| IBIS file stm32u535_545_ufbga100_smps.ibs
[IBIS ver] 4.2
[File name] stm32u535_545_ufbga100_smps.ibs
[File Rev] rev1.0
[Date]  11-09-2023
[Source] Data Created at STMicroelectronics
[Notes]  File originated from ELDO simulations.
[Disclaimer]  This information is for modeling purpose only and is
   not guaranteed. The information is subject to change without
   notice.
[Copyright] Copyright 2023 STMicroelectronics Inc.
|   Component stm32u535_545_ufbga100_smps
[Component] stm32u535_545_ufbga100_smps
[Manufacturer] STMicroelectronics
[Package]
| variable   typ   min   max
R_pkg  0  NA  NA
L_pkg  0  NA  NA
C_pkg  0  NA  NA
[Pin]   signal_name   model_name
A1  PB9  io8_100m_hslv_i2c_ft
A2  PE0  io8_100m_hslv_ft
A3  PH3-BOOT0  io8_100m_ft
A4  PB7  io8_166m_hslv_i2c_ft
A5  PB6  io8_100m_i2c_ft
A6  PB4  io8_100m_i2c_ft
A7  PD7  io8_100m_hslv_ft
A8  PD5  io8_100m_hslv_ft
A9  PD4  io8_100m_hslv_ft
A10  PD2  io8_100m_hslv_ft
A11  PD0  io8_100m_hslv_ft
A12  PC10  io8_100m_hslv_ft
B1  PE2  io8_100m_hslv_ft
B2  PE3  io8_100m_hslv_tamp_ft
B3  PE4  io8_100m_hslv_tamp_ft
B4  PB8  io8_100m_hslv_i2c_ft
B5  PB5  io8_166m_hslv_ft
B6  PB3  io8_100m_i2c_ft
B7  VDD  power
B8  PD6  io8_166m_hslv_ft
B9  PD3  io8_166m_hslv_ft
B10  PD1  io8_100m_hslv_ft
B11  PC11  io8_100m_hslv_ft
B12  PA15  io8_100m_ft
C1  VBAT  power
C2  PE6  io8_100m_hslv_tamp_ft
C3  VDD  power
C4  VSS  gnd
C5  VDD11  nc
C8  VSS  gnd
C9  PC12  io8_166m_hslv_ft
C10  VDD  power
C11  PA14  io8_100m_ft
C12  PA13  io8_100m_ft
D1  PC14-OSC32_IN  io8_100m_tamp_ft
D2  PC15-OSC32_OUT  io8_100m_tamp_ft
D3  PE5  io8_100m_hslv_tamp_ft
D10  VSS  gnd
D11  PA12  io8_usb_ft
D12  PA11  io8_usb_ft
E1  PH0-OSC_IN  io8_100m_ft
E2  PH1-OSC_OUT  io8_100m_ft
E3  PC13  io8_100m_ft_v33
E10  VDDUSB  power
E11  PA9  io8_100m_ft
E12  PA10  io8_100m_ft
F1  NRST  nc
F2  PC0  io8_100m_hslv_i2c_ft
F11  PC9  io8_100m_hslv_ft
F12  PA8  io8_166m_hslv_ft
G1  PC1  io8_166m_hslv_i2c_ft
G2  PC2  io8_100m_hslv_ft
G11  PC7  io8_100m_hslv_ft
G12  PC8  io8_100m_hslv_ft
H1  VREFP  nc
H2  VSSA  nc
H3  PC3  io8_100m_hslv_ft
H10  PD12  io8_100m_hslv_i2c_ft
H11  PD15  io8_100m_hslv_ft
H12  PC6  io8_100m_hslv_ft
J1  VDDA  power
J2  PA1  io8_100m_hslv_tamp_ft
J3  PA0  io8_100m_hslv_tamp_ft
J10  PD8  io8_100m_hslv_ft
J11  PD13  io8_100m_hslv_i2c_ft
J12  PD14  io8_100m_hslv_ft
K1  PA2  io8_100m_hslv_ft
K2  PA3  io8_166m_hslv_ft
K3  VSS  gnd
K4  VDD  power
K5  PE7  io8_100m_hslv_ft
K8  PB11  io8_100m_hslv_i2c_ft
K9  VDD11  nc
K10  VDD  power
K11  PD9  io8_100m_hslv_ft
K12  PD11  io8_100m_hslv_ft
L1  PA4  io8_100m_hslv_ft
L2  PA5  io8_100m_ft
L3  PB0  io8_100m_hslv_ft
L4  PB2  io8_100m_hslv_tamp_ft
L5  PE9  io8_166m_hslv_ft
L6  PE11  io8_100m_hslv_ft
L7  PE13  io8_100m_hslv_ft
L8  PE15  io8_100m_hslv_ft
L9  VSSSMPS  nc
L10  VSS  gnd
L11  PB13  io8_100m_i2c_ft
L12  PD10  io8_100m_hslv_ft
M1  PA6  io8_100m_hslv_ft
M2  PA7  io8_100m_hslv_i2c_ft
M3  PB1  io8_100m_hslv_ft
M4  PE8  io8_100m_hslv_ft
M5  PE10  io8_166m_hslv_ft
M6  PE12  io8_100m_hslv_ft
M7  PE14  io8_100m_hslv_ft
M8  PB10  io8_166m_hslv_i2c_ft
M9  VLXSMPS  nc
M10  VDDSMPS  nc
M11  PB14  io8_100m_i2c_ft
M12  PB15  io8_100m_ft
[Package Model]   455-ufbga-7x7-100-smps-100mhz-230421
[Pin Mapping]   pulldown_ref   pullup_ref   | Comment
A1  gndio  vddiom
A2  gndio  vddiom
A3  gndio  vddiom
A4  gndio  vddiom
A5  gndio  vddiom
A6  gndio  vddiom
A7  gndio  vddiom
A8  gndio  vddiom
A9  gndio  vddiom
A10  gndio  vddiom
A11  gndio  vddiom
A12  gndio  vddiom
B1  gndio  vddiom
B2  gndio  vddiom
B3  gndio  vddiom
B4  gndio  vddiom
B5  gndio  vddiom
B6  gndio  vddiom
B7  nc  vddiom
B8  gndio  vddiom
B9  gndio  vddiom
B10  gndio  vddiom
B11  gndio  vddiom
B12  gndio  vddiom
C1  nc  vsw
C2  gndio  vddiom
C3  nc  vddiom
C4  gndio  nc
C5  nc  nc
C8  gndio  nc
C9  gndio  vddiom
C10  nc  vddiom
C11  gndio  vddiom
C12  gndio  vddiom  | Depending on IO usage
| C12  gndio  vddusb  | Depending on IO usage
D1  gndio  vddiom  | Depending on IO usage
| D1  gndio  vsw  | Depending on IO usage
D2  gndio  vddiom  | Depending on IO usage
| D2  gndio  vsw  | Depending on IO usage
D3  gndio  vddiom
D10  gndio  nc
D11  gndio  vddiom  | Depending on IO usage
| D11  gndio  vddusb  | Depending on IO usage
D12  gndio  vddiom  | Depending on IO usage
| D12  gndio  vddusb  | Depending on IO usage
E1  gndio  vddiom
E2  gndio  vddiom
E3  gndio  vddiom  | Depending on IO usage
| E3  gndio  vsw  | Depending on IO usage
E10  nc  vddusb
E11  gndio  vddiom  | Depending on IO usage
| E11  gndio  vddusb  | Depending on IO usage
E12  gndio  vddiom  | Depending on IO usage
| E12  gndio  vddusb  | Depending on IO usage
F1  nc   nc
F2  gndio  vddiom
F11  gndio  vddiom
F12  gndio  vddiom
G1  gndio  vddiom
G2  gndio  vddiom
G11  gndio  vddiom
G12  gndio  vddiom
H1  nc  nc
H2  nc  nc
H3  gndio  vddiom
H10  gndio  vddiom
H11  gndio  vddiom
H12  gndio  vddiom
J1  nc  vddiom
J2  gndio  vddiom
J3  gndio  vddiom
J10  gndio  vddiom
J11  gndio  vddiom
J12  gndio  vddiom
K1  gndio  vddiom
K2  gndio  vddiom
K3  gndio  nc
K4  nc  vddiom
K5  gndio  vddiom
K8  gndio  vddiom
K9  nc  nc
K10  nc  vddiom
K11  gndio  vddiom
K12  gndio  vddiom
L1  gndio  vddiom
L2  gndio  vddiom
L3  gndio  vddiom
L4  gndio  vddiom
L5  gndio  vddiom
L6  gndio  vddiom
L7  gndio  vddiom
L8  gndio  vddiom
L9  nc  nc
L10  gndio  nc
L11  gndio  vddiom
L12  gndio  vddiom
M1  gndio  vddiom
M2  gndio  vddiom
M3  gndio  vddiom
M4  gndio  vddiom
M5  gndio  vddiom
M6  gndio  vddiom
M7  gndio  vddiom
M8  gndio  vddiom
M9  nc  nc
M10  nc  nc
M11  gndio  vddiom
M12  gndio  vddiom
[Model Selector] io8_100m_ft
io8_100m_ft_hs_1v2  "IO8_FT 100MHz high speed @ 1.2V"
io8_100m_ft_fs_1v2  "IO8_FT 100MHz fast speed @ 1.2V"
io8_100m_ft_fs_pd_1v2  "IO8_FT 100MHz fast speed @ 1.2V pulldown"
io8_100m_ft_ms_1v2  "IO8_FT 100MHz med speed @ 1.2V"
io8_100m_ft_ms_pd_1v2  "IO8_FT 100MHz med speed @ 1.2V pulldown"
io8_100m_ft_ls_1v2  "IO8_FT 100MHz low speed @ 1.2V"
io8_100m_ft_ls_pd_1v2  "IO8_FT 100MHz low speed @ 1.2V pulldown"
io8_100m_ft_hs_1v8  "IO8_FT 100MHz high speed @ 1.8V"
io8_100m_ft_hs_pd_1v8  "IO8_FT 100MHz high speed @ 1.8V pulldown"
io8_100m_ft_fs_1v8  "IO8_FT 100MHz fast speed @ 1.8V"
io8_100m_ft_fs_pd_1v8  "IO8_FT 100MHz fast speed @ 1.8V pulldown"
io8_100m_ft_ms_1v8  "IO8_FT 100MHz med speed @ 1.8V"
io8_100m_ft_ms_pd_1v8  "IO8_FT 100MHz med speed @ 1.8V pulldown"
io8_100m_ft_ls_1v8  "IO8_FT 100MHz low speed @ 1.8V"
io8_100m_ft_ls_pd_1v8  "IO8_FT 100MHz low speed @ 1.8V pulldown"
io8_100m_ft_hs_3v3  "IO8_FT 100MHz high speed @ 3.3V"
io8_100m_ft_hs_pd_3v3  "IO8_FT 100MHz high speed @ 3.3V pulldown"
io8_100m_ft_fs_3v3  "IO8_FT 100MHz fast speed @ 3.3V"
io8_100m_ft_fs_pd_3v3  "IO8_FT 100MHz fast speed @ 3.3V pulldown"
io8_100m_ft_ms_3v3  "IO8_FT 100MHz med speed @ 3.3V"
io8_100m_ft_ms_pd_3v3  "IO8_FT 100MHz med speed @ 3.3V pulldown"
io8_100m_ft_ls_3v3  "IO8_FT 100MHz low speed @ 3.3V"
io8_100m_ft_ls_pd_3v3  "IO8_FT 100MHz low speed @ 3.3V pulldown"
[Model Selector] io8_100m_hslv_ft
io8_100m_ft_hs_1v2  "IO8_FT 100MHz high speed @ 1.2V"
io8_100m_ft_hs_pu_1v2  "IO8_FT 100MHz high speed @ 1.2V pullup"
io8_100m_ft_hs_pd_1v2  "IO8_FT 100MHz high speed @ 1.2V pulldown"
io8_100m_ft_fs_1v2  "IO8_FT 100MHz fast speed @ 1.2V"
io8_100m_ft_fs_pu_1v2  "IO8_FT 100MHz fast speed @ 1.2V pullup"
io8_100m_ft_fs_pd_1v2  "IO8_FT 100MHz fast speed @ 1.2V pulldown"
io8_100m_ft_ms_1v2  "IO8_FT 100MHz med speed @ 1.2V"
io8_100m_ft_ms_pu_1v2  "IO8_FT 100MHz med speed @ 1.2V pullup"
io8_100m_ft_ms_pd_1v2  "IO8_FT 100MHz med speed @ 1.2V pulldown"
io8_100m_ft_ls_1v2  "IO8_FT 100MHz low speed @ 1.2V"
io8_100m_ft_ls_pu_1v2  "IO8_FT 100MHz low speed @ 1.2V pullup"
io8_100m_ft_ls_pd_1v2  "IO8_FT 100MHz low speed @ 1.2V pulldown"
io8_100m_ft_hs_1v8  "IO8_FT 100MHz high speed @ 1.8V"
io8_100m_ft_hs_pu_1v8  "IO8_FT 100MHz high speed @ 1.8V pullup"
io8_100m_ft_hs_pd_1v8  "IO8_FT 100MHz high speed @ 1.8V pulldown"
io8_100m_ft_fs_1v8  "IO8_FT 100MHz fast speed @ 1.8V"
io8_100m_ft_fs_pu_1v8  "IO8_FT 100MHz fast speed @ 1.8V pullup"
io8_100m_ft_fs_pd_1v8  "IO8_FT 100MHz fast speed @ 1.8V pulldown"
io8_100m_ft_ms_1v8  "IO8_FT 100MHz med speed @ 1.8V"
io8_100m_ft_ms_pu_1v8  "IO8_FT 100MHz med speed @ 1.8V pullup"
io8_100m_ft_ms_pd_1v8  "IO8_FT 100MHz med speed @ 1.8V pulldown"
io8_100m_ft_ls_1v8  "IO8_FT 100MHz low speed @ 1.8V"
io8_100m_ft_ls_pu_1v8  "IO8_FT 100MHz low speed @ 1.8V pullup"
io8_100m_ft_ls_pd_1v8  "IO8_FT 100MHz low speed @ 1.8V pulldown"
io8_100m_ft_hs_3v3  "IO8_FT 100MHz high speed @ 3.3V"
io8_100m_ft_hs_pu_3v3  "IO8_FT 100MHz high speed @ 3.3V pullup"
io8_100m_ft_hs_pd_3v3  "IO8_FT 100MHz high speed @ 3.3V pulldown"
io8_100m_ft_fs_3v3  "IO8_FT 100MHz fast speed @ 3.3V"
io8_100m_ft_fs_pu_3v3  "IO8_FT 100MHz fast speed @ 3.3V pullup"
io8_100m_ft_fs_pd_3v3  "IO8_FT 100MHz fast speed @ 3.3V pulldown"
io8_100m_ft_ms_3v3  "IO8_FT 100MHz med speed @ 3.3V"
io8_100m_ft_ms_pu_3v3  "IO8_FT 100MHz med speed @ 3.3V pullup"
io8_100m_ft_ms_pd_3v3  "IO8_FT 100MHz med speed @ 3.3V pulldown"
io8_100m_ft_ls_3v3  "IO8_FT 100MHz low speed @ 3.3V"
io8_100m_ft_ls_pu_3v3  "IO8_FT 100MHz low speed @ 3.3V pullup"
io8_100m_ft_ls_pd_3v3  "IO8_FT 100MHz low speed @ 3.3V pulldown"
io8_100m_hslv_ft_hs_1v2  "IO8_FT 100MHz HSLV high speed @ 1.2V"
io8_100m_hslv_ft_hs_pu_1v2  "IO8_FT 100MHz HSLV high speed @ 1.2V pullup"
io8_100m_hslv_ft_hs_pd_1v2  "IO8_FT 100MHz HSLV high speed @ 1.2V pulldown"
io8_100m_hslv_ft_fs_1v2  "IO8_FT 100MHz HSLV fast speed @ 1.2V"
io8_100m_hslv_ft_fs_pu_1v2  "IO8_FT 100MHz HSLV fast speed @ 1.2V pullup"
io8_100m_hslv_ft_fs_pd_1v2  "IO8_FT 100MHz HSLV fast speed @ 1.2V pulldown"
io8_100m_hslv_ft_ms_1v2  "IO8_FT 100MHz HSLV med speed @ 1.2V"
io8_100m_hslv_ft_ms_pu_1v2  "IO8_FT 100MHz HSLV med speed @ 1.2V pullup"
io8_100m_hslv_ft_ms_pd_1v2  "IO8_FT 100MHz HSLV med speed @ 1.2V pulldown"
io8_100m_hslv_ft_ls_1v2  "IO8_FT 100MHz HSLV low speed @ 1.2V"
io8_100m_hslv_ft_ls_pu_1v2  "IO8_FT 100MHz HSLV low speed @ 1.2V pullup"
io8_100m_hslv_ft_ls_pd_1v2  "IO8_FT 100MHz HSLV low speed @ 1.2V pulldown"
io8_100m_hslv_ft_hs_1v8  "IO8_FT 100MHz HSLV high speed @ 1.8V"
io8_100m_hslv_ft_hs_pu_1v8  "IO8_FT 100MHz HSLV high speed @ 1.8V pullup"
io8_100m_hslv_ft_hs_pd_1v8  "IO8_FT 100MHz HSLV high speed @ 1.8V pulldown"
io8_100m_hslv_ft_fs_1v8  "IO8_FT 100MHz HSLV fast speed @ 1.8V"
io8_100m_hslv_ft_fs_pu_1v8  "IO8_FT 100MHz HSLV fast speed @ 1.8V pullup"
io8_100m_hslv_ft_fs_pd_1v8  "IO8_FT 100MHz HSLV fast speed @ 1.8V pulldown"
io8_100m_hslv_ft_ms_1v8  "IO8_FT 100MHz HSLV med speed @ 1.8V"
io8_100m_hslv_ft_ms_pu_1v8  "IO8_FT 100MHz HSLV med speed @ 1.8V pullup"
io8_100m_hslv_ft_ms_pd_1v8  "IO8_FT 100MHz HSLV med speed @ 1.8V pulldown"
io8_100m_hslv_ft_ls_1v8  "IO8_FT 100MHz HSLV low speed @ 1.8V"
io8_100m_hslv_ft_ls_pu_1v8  "IO8_FT 100MHz HSLV low speed @ 1.8V pullup"
io8_100m_hslv_ft_ls_pd_1v8  "IO8_FT 100MHz HSLV low speed @ 1.8V pulldown"
io8_100m_hslv_ft_hs_2v5  "IO8_FT 100MHz HSLV high speed @ 2.5V"
io8_100m_hslv_ft_hs_pu_2v5  "IO8_FT 100MHz HSLV high speed @ 2.5V pullup"
io8_100m_hslv_ft_hs_pd_2v5  "IO8_FT 100MHz HSLV high speed @ 2.5V pulldown"
io8_100m_hslv_ft_fs_2v5  "IO8_FT 100MHz HSLV fast speed @ 2.5V"
io8_100m_hslv_ft_fs_pu_2v5  "IO8_FT 100MHz HSLV fast speed @ 2.5V pullup"
io8_100m_hslv_ft_fs_pd_2v5  "IO8_FT 100MHz HSLV fast speed @ 2.5V pulldown"
io8_100m_hslv_ft_ms_2v5  "IO8_FT 100MHz HSLV med speed @ 2.5V"
io8_100m_hslv_ft_ms_pu_2v5  "IO8_FT 100MHz HSLV med speed @ 2.5V pullup"
io8_100m_hslv_ft_ms_pd_2v5  "IO8_FT 100MHz HSLV med speed @ 2.5V pulldown"
io8_100m_hslv_ft_ls_2v5  "IO8_FT 100MHz HSLV low speed @ 2.5V"
io8_100m_hslv_ft_ls_pu_2v5  "IO8_FT 100MHz HSLV low speed @ 2.5V pullup"
io8_100m_hslv_ft_ls_pd_2v5  "IO8_FT 100MHz HSLV low speed @ 2.5V pulldown"
[Model Selector] io8_100m_hslv_i2c_ft
io8_100m_ft_hs_1v2  "IO8_FT 100MHz high speed @ 1.2V"
io8_100m_ft_hs_pu_1v2  "IO8_FT 100MHz high speed @ 1.2V pullup"
io8_100m_ft_hs_pd_1v2  "IO8_FT 100MHz high speed @ 1.2V pulldown"
io8_100m_ft_fs_1v2  "IO8_FT 100MHz fast speed @ 1.2V"
io8_100m_ft_fs_pu_1v2  "IO8_FT 100MHz fast speed @ 1.2V pullup"
io8_100m_ft_fs_pd_1v2  "IO8_FT 100MHz fast speed @ 1.2V pulldown"
io8_100m_ft_ms_1v2  "IO8_FT 100MHz med speed @ 1.2V"
io8_100m_ft_ms_pu_1v2  "IO8_FT 100MHz med speed @ 1.2V pullup"
io8_100m_ft_ms_pd_1v2  "IO8_FT 100MHz med speed @ 1.2V pulldown"
io8_100m_ft_ls_1v2  "IO8_FT 100MHz low speed @ 1.2V"
io8_100m_ft_ls_pu_1v2  "IO8_FT 100MHz low speed @ 1.2V pullup"
io8_100m_ft_ls_pd_1v2  "IO8_FT 100MHz low speed @ 1.2V pulldown"
io8_100m_ft_hs_1v8  "IO8_FT 100MHz high speed @ 1.8V"
io8_100m_ft_hs_pu_1v8  "IO8_FT 100MHz high speed @ 1.8V pullup"
io8_100m_ft_hs_pd_1v8  "IO8_FT 100MHz high speed @ 1.8V pulldown"
io8_100m_ft_fs_1v8  "IO8_FT 100MHz fast speed @ 1.8V"
io8_100m_ft_fs_pu_1v8  "IO8_FT 100MHz fast speed @ 1.8V pullup"
io8_100m_ft_fs_pd_1v8  "IO8_FT 100MHz fast speed @ 1.8V pulldown"
io8_100m_ft_ms_1v8  "IO8_FT 100MHz med speed @ 1.8V"
io8_100m_ft_ms_pu_1v8  "IO8_FT 100MHz med speed @ 1.8V pullup"
io8_100m_ft_ms_pd_1v8  "IO8_FT 100MHz med speed @ 1.8V pulldown"
io8_100m_ft_ls_1v8  "IO8_FT 100MHz low speed @ 1.8V"
io8_100m_ft_ls_pu_1v8  "IO8_FT 100MHz low speed @ 1.8V pullup"
io8_100m_ft_ls_pd_1v8  "IO8_FT 100MHz low speed @ 1.8V pulldown"
io8_100m_ft_hs_3v3  "IO8_FT 100MHz high speed @ 3.3V"
io8_100m_ft_hs_pu_3v3  "IO8_FT 100MHz high speed @ 3.3V pullup"
io8_100m_ft_hs_pd_3v3  "IO8_FT 100MHz high speed @ 3.3V pulldown"
io8_100m_ft_fs_3v3  "IO8_FT 100MHz fast speed @ 3.3V"
io8_100m_ft_fs_pu_3v3  "IO8_FT 100MHz fast speed @ 3.3V pullup"
io8_100m_ft_fs_pd_3v3  "IO8_FT 100MHz fast speed @ 3.3V pulldown"
io8_100m_ft_ms_3v3  "IO8_FT 100MHz med speed @ 3.3V"
io8_100m_ft_ms_pu_3v3  "IO8_FT 100MHz med speed @ 3.3V pullup"
io8_100m_ft_ms_pd_3v3  "IO8_FT 100MHz med speed @ 3.3V pulldown"
io8_100m_ft_ls_3v3  "IO8_FT 100MHz low speed @ 3.3V"
io8_100m_ft_ls_pu_3v3  "IO8_FT 100MHz low speed @ 3.3V pullup"
io8_100m_ft_ls_pd_3v3  "IO8_FT 100MHz low speed @ 3.3V pulldown"
io8_100m_hslv_ft_hs_1v2  "IO8_FT 100MHz HSLV high speed @ 1.2V"
io8_100m_hslv_ft_hs_pu_1v2  "IO8_FT 100MHz HSLV high speed @ 1.2V pullup"
io8_100m_hslv_ft_hs_pd_1v2  "IO8_FT 100MHz HSLV high speed @ 1.2V pulldown"
io8_100m_hslv_ft_fs_1v2  "IO8_FT 100MHz HSLV fast speed @ 1.2V"
io8_100m_hslv_ft_fs_pu_1v2  "IO8_FT 100MHz HSLV fast speed @ 1.2V pullup"
io8_100m_hslv_ft_fs_pd_1v2  "IO8_FT 100MHz HSLV fast speed @ 1.2V pulldown"
io8_100m_hslv_ft_ms_1v2  "IO8_FT 100MHz HSLV med speed @ 1.2V"
io8_100m_hslv_ft_ms_pu_1v2  "IO8_FT 100MHz HSLV med speed @ 1.2V pullup"
io8_100m_hslv_ft_ms_pd_1v2  "IO8_FT 100MHz HSLV med speed @ 1.2V pulldown"
io8_100m_hslv_ft_ls_1v2  "IO8_FT 100MHz HSLV low speed @ 1.2V"
io8_100m_hslv_ft_ls_pu_1v2  "IO8_FT 100MHz HSLV low speed @ 1.2V pullup"
io8_100m_hslv_ft_ls_pd_1v2  "IO8_FT 100MHz HSLV low speed @ 1.2V pulldown"
io8_100m_hslv_ft_hs_1v8  "IO8_FT 100MHz HSLV high speed @ 1.8V"
io8_100m_hslv_ft_hs_pu_1v8  "IO8_FT 100MHz HSLV high speed @ 1.8V pullup"
io8_100m_hslv_ft_hs_pd_1v8  "IO8_FT 100MHz HSLV high speed @ 1.8V pulldown"
io8_100m_hslv_ft_fs_1v8  "IO8_FT 100MHz HSLV fast speed @ 1.8V"
io8_100m_hslv_ft_fs_pu_1v8  "IO8_FT 100MHz HSLV fast speed @ 1.8V pullup"
io8_100m_hslv_ft_fs_pd_1v8  "IO8_FT 100MHz HSLV fast speed @ 1.8V pulldown"
io8_100m_hslv_ft_ms_1v8  "IO8_FT 100MHz HSLV med speed @ 1.8V"
io8_100m_hslv_ft_ms_pu_1v8  "IO8_FT 100MHz HSLV med speed @ 1.8V pullup"
io8_100m_hslv_ft_ms_pd_1v8  "IO8_FT 100MHz HSLV med speed @ 1.8V pulldown"
io8_100m_hslv_ft_ls_1v8  "IO8_FT 100MHz HSLV low speed @ 1.8V"
io8_100m_hslv_ft_ls_pu_1v8  "IO8_FT 100MHz HSLV low speed @ 1.8V pullup"
io8_100m_hslv_ft_ls_pd_1v8  "IO8_FT 100MHz HSLV low speed @ 1.8V pulldown"
io8_100m_hslv_ft_hs_2v5  "IO8_FT 100MHz HSLV high speed @ 2.5V"
io8_100m_hslv_ft_hs_pu_2v5  "IO8_FT 100MHz HSLV high speed @ 2.5V pullup"
io8_100m_hslv_ft_hs_pd_2v5  "IO8_FT 100MHz HSLV high speed @ 2.5V pulldown"
io8_100m_hslv_ft_fs_2v5  "IO8_FT 100MHz HSLV fast speed @ 2.5V"
io8_100m_hslv_ft_fs_pu_2v5  "IO8_FT 100MHz HSLV fast speed @ 2.5V pullup"
io8_100m_hslv_ft_fs_pd_2v5  "IO8_FT 100MHz HSLV fast speed @ 2.5V pulldown"
io8_100m_hslv_ft_ms_2v5  "IO8_FT 100MHz HSLV med speed @ 2.5V"
io8_100m_hslv_ft_ms_pu_2v5  "IO8_FT 100MHz HSLV med speed @ 2.5V pullup"
io8_100m_hslv_ft_ms_pd_2v5  "IO8_FT 100MHz HSLV med speed @ 2.5V pulldown"
io8_100m_hslv_ft_ls_2v5  "IO8_FT 100MHz HSLV low speed @ 2.5V"
io8_100m_hslv_ft_ls_pu_2v5  "IO8_FT 100MHz HSLV low speed @ 2.5V pullup"
io8_100m_hslv_ft_ls_pd_2v5  "IO8_FT 100MHz HSLV low speed @ 2.5V pulldown"
[Model Selector] io8_100m_hslv_tamp_ft
io8_100m_ft_hs_1v2  "IO8_FT 100MHz high speed @ 1.2V"
io8_100m_ft_hs_pu_1v2  "IO8_FT 100MHz high speed @ 1.2V pullup"
io8_100m_ft_hs_pd_1v2  "IO8_FT 100MHz high speed @ 1.2V pulldown"
io8_100m_ft_fs_1v2  "IO8_FT 100MHz fast speed @ 1.2V"
io8_100m_ft_fs_pu_1v2  "IO8_FT 100MHz fast speed @ 1.2V pullup"
io8_100m_ft_fs_pd_1v2  "IO8_FT 100MHz fast speed @ 1.2V pulldown"
io8_100m_ft_ms_1v2  "IO8_FT 100MHz med speed @ 1.2V"
io8_100m_ft_ms_pu_1v2  "IO8_FT 100MHz med speed @ 1.2V pullup"
io8_100m_ft_ms_pd_1v2  "IO8_FT 100MHz med speed @ 1.2V pulldown"
io8_100m_ft_ls_1v2  "IO8_FT 100MHz low speed @ 1.2V"
io8_100m_ft_ls_pu_1v2  "IO8_FT 100MHz low speed @ 1.2V pullup"
io8_100m_ft_ls_pd_1v2  "IO8_FT 100MHz low speed @ 1.2V pulldown"
io8_100m_ft_hs_1v8  "IO8_FT 100MHz high speed @ 1.8V"
io8_100m_ft_hs_pu_1v8  "IO8_FT 100MHz high speed @ 1.8V pullup"
io8_100m_ft_hs_pd_1v8  "IO8_FT 100MHz high speed @ 1.8V pulldown"
io8_100m_ft_fs_1v8  "IO8_FT 100MHz fast speed @ 1.8V"
io8_100m_ft_fs_pu_1v8  "IO8_FT 100MHz fast speed @ 1.8V pullup"
io8_100m_ft_fs_pd_1v8  "IO8_FT 100MHz fast speed @ 1.8V pulldown"
io8_100m_ft_ms_1v8  "IO8_FT 100MHz med speed @ 1.8V"
io8_100m_ft_ms_pu_1v8  "IO8_FT 100MHz med speed @ 1.8V pullup"
io8_100m_ft_ms_pd_1v8  "IO8_FT 100MHz med speed @ 1.8V pulldown"
io8_100m_ft_ls_1v8  "IO8_FT 100MHz low speed @ 1.8V"
io8_100m_ft_ls_pu_1v8  "IO8_FT 100MHz low speed @ 1.8V pullup"
io8_100m_ft_ls_pd_1v8  "IO8_FT 100MHz low speed @ 1.8V pulldown"
io8_100m_ft_hs_3v3  "IO8_FT 100MHz high speed @ 3.3V"
io8_100m_ft_hs_pu_3v3  "IO8_FT 100MHz high speed @ 3.3V pullup"
io8_100m_ft_hs_pd_3v3  "IO8_FT 100MHz high speed @ 3.3V pulldown"
io8_100m_ft_fs_3v3  "IO8_FT 100MHz fast speed @ 3.3V"
io8_100m_ft_fs_pu_3v3  "IO8_FT 100MHz fast speed @ 3.3V pullup"
io8_100m_ft_fs_pd_3v3  "IO8_FT 100MHz fast speed @ 3.3V pulldown"
io8_100m_ft_ms_3v3  "IO8_FT 100MHz med speed @ 3.3V"
io8_100m_ft_ms_pu_3v3  "IO8_FT 100MHz med speed @ 3.3V pullup"
io8_100m_ft_ms_pd_3v3  "IO8_FT 100MHz med speed @ 3.3V pulldown"
io8_100m_ft_ls_3v3  "IO8_FT 100MHz low speed @ 3.3V"
io8_100m_ft_ls_pu_3v3  "IO8_FT 100MHz low speed @ 3.3V pullup"
io8_100m_ft_ls_pd_3v3  "IO8_FT 100MHz low speed @ 3.3V pulldown"
io8_100m_hslv_ft_hs_1v2  "IO8_FT 100MHz HSLV high speed @ 1.2V"
io8_100m_hslv_ft_hs_pu_1v2  "IO8_FT 100MHz HSLV high speed @ 1.2V pullup"
io8_100m_hslv_ft_hs_pd_1v2  "IO8_FT 100MHz HSLV high speed @ 1.2V pulldown"
io8_100m_hslv_ft_fs_1v2  "IO8_FT 100MHz HSLV fast speed @ 1.2V"
io8_100m_hslv_ft_fs_pu_1v2  "IO8_FT 100MHz HSLV fast speed @ 1.2V pullup"
io8_100m_hslv_ft_fs_pd_1v2  "IO8_FT 100MHz HSLV fast speed @ 1.2V pulldown"
io8_100m_hslv_ft_ms_1v2  "IO8_FT 100MHz HSLV med speed @ 1.2V"
io8_100m_hslv_ft_ms_pu_1v2  "IO8_FT 100MHz HSLV med speed @ 1.2V pullup"
io8_100m_hslv_ft_ms_pd_1v2  "IO8_FT 100MHz HSLV med speed @ 1.2V pulldown"
io8_100m_hslv_ft_ls_1v2  "IO8_FT 100MHz HSLV low speed @ 1.2V"
io8_100m_hslv_ft_ls_pu_1v2  "IO8_FT 100MHz HSLV low speed @ 1.2V pullup"
io8_100m_hslv_ft_ls_pd_1v2  "IO8_FT 100MHz HSLV low speed @ 1.2V pulldown"
io8_100m_hslv_ft_hs_1v8  "IO8_FT 100MHz HSLV high speed @ 1.8V"
io8_100m_hslv_ft_hs_pu_1v8  "IO8_FT 100MHz HSLV high speed @ 1.8V pullup"
io8_100m_hslv_ft_hs_pd_1v8  "IO8_FT 100MHz HSLV high speed @ 1.8V pulldown"
io8_100m_hslv_ft_fs_1v8  "IO8_FT 100MHz HSLV fast speed @ 1.8V"
io8_100m_hslv_ft_fs_pu_1v8  "IO8_FT 100MHz HSLV fast speed @ 1.8V pullup"
io8_100m_hslv_ft_fs_pd_1v8  "IO8_FT 100MHz HSLV fast speed @ 1.8V pulldown"
io8_100m_hslv_ft_ms_1v8  "IO8_FT 100MHz HSLV med speed @ 1.8V"
io8_100m_hslv_ft_ms_pu_1v8  "IO8_FT 100MHz HSLV med speed @ 1.8V pullup"
io8_100m_hslv_ft_ms_pd_1v8  "IO8_FT 100MHz HSLV med speed @ 1.8V pulldown"
io8_100m_hslv_ft_ls_1v8  "IO8_FT 100MHz HSLV low speed @ 1.8V"
io8_100m_hslv_ft_ls_pu_1v8  "IO8_FT 100MHz HSLV low speed @ 1.8V pullup"
io8_100m_hslv_ft_ls_pd_1v8  "IO8_FT 100MHz HSLV low speed @ 1.8V pulldown"
io8_100m_hslv_ft_hs_2v5  "IO8_FT 100MHz HSLV high speed @ 2.5V"
io8_100m_hslv_ft_hs_pu_2v5  "IO8_FT 100MHz HSLV high speed @ 2.5V pullup"
io8_100m_hslv_ft_hs_pd_2v5  "IO8_FT 100MHz HSLV high speed @ 2.5V pulldown"
io8_100m_hslv_ft_fs_2v5  "IO8_FT 100MHz HSLV fast speed @ 2.5V"
io8_100m_hslv_ft_fs_pu_2v5  "IO8_FT 100MHz HSLV fast speed @ 2.5V pullup"
io8_100m_hslv_ft_fs_pd_2v5  "IO8_FT 100MHz HSLV fast speed @ 2.5V pulldown"
io8_100m_hslv_ft_ms_2v5  "IO8_FT 100MHz HSLV med speed @ 2.5V"
io8_100m_hslv_ft_ms_pu_2v5  "IO8_FT 100MHz HSLV med speed @ 2.5V pullup"
io8_100m_hslv_ft_ms_pd_2v5  "IO8_FT 100MHz HSLV med speed @ 2.5V pulldown"
io8_100m_hslv_ft_ls_2v5  "IO8_FT 100MHz HSLV low speed @ 2.5V"
io8_100m_hslv_ft_ls_pu_2v5  "IO8_FT 100MHz HSLV low speed @ 2.5V pullup"
io8_100m_hslv_ft_ls_pd_2v5  "IO8_FT 100MHz HSLV low speed @ 2.5V pulldown"
io8_ft_v33_hs_1v2  "IO8_FT_V33 high speed @ 1.2V"
io8_ft_v33_hs_pu_1v2  "IO8_FT_V33 high speed @ 1.2V pullup"
io8_ft_v33_hs_pd_1v2  "IO8_FT_V33 high speed @ 1.2V pulldown"
io8_ft_v33_fs_1v2  "IO8_FT_V33 fast speed @ 1.2V"
io8_ft_v33_fs_pu_1v2  "IO8_FT_V33 fast speed @ 1.2V pullup"
io8_ft_v33_fs_pd_1v2  "IO8_FT_V33 fast speed @ 1.2V pulldown"
io8_ft_v33_ms_1v2  "IO8_FT_V33 med speed @ 1.2V"
io8_ft_v33_ms_pu_1v2  "IO8_FT_V33 med speed @ 1.2V pullup"
io8_ft_v33_ms_pd_1v2  "IO8_FT_V33 med speed @ 1.2V pulldown"
io8_ft_v33_ls_1v2  "IO8_FT_V33 low speed @ 1.2V"
io8_ft_v33_ls_pu_1v2  "IO8_FT_V33 low speed @ 1.2V pullup"
io8_ft_v33_ls_pd_1v2  "IO8_FT_V33 low speed @ 1.2V pulldown"
io8_ft_v33_hs_1v8  "IO8_FT_V33 high speed @ 1.8V"
io8_ft_v33_hs_pu_1v8  "IO8_FT_V33 high speed @ 1.8V pullup"
io8_ft_v33_hs_pd_1v8  "IO8_FT_V33 high speed @ 1.8V pulldown"
io8_ft_v33_fs_1v8  "IO8_FT_V33 fast speed @ 1.8V"
io8_ft_v33_fs_pu_1v8  "IO8_FT_V33 fast speed @ 1.8V pullup"
io8_ft_v33_fs_pd_1v8  "IO8_FT_V33 fast speed @ 1.8V pulldown"
io8_ft_v33_ms_1v8  "IO8_FT_V33 med speed @ 1.8V"
io8_ft_v33_ms_pu_1v8  "IO8_FT_V33 med speed @ 1.8V pullup"
io8_ft_v33_ms_pd_1v8  "IO8_FT_V33 med speed @ 1.8V pulldown"
io8_ft_v33_ls_1v8  "IO8_FT_V33 low speed @ 1.8V"
io8_ft_v33_ls_pu_1v8  "IO8_FT_V33 low speed @ 1.8V pullup"
io8_ft_v33_ls_pd_1v8  "IO8_FT_V33 low speed @ 1.8V pulldown"
io8_ft_v33_hs_3v3  "IO8_FT_V33 high speed @ 3.3V"
io8_ft_v33_hs_pu_3v3  "IO8_FT_V33 high speed @ 3.3V pullup"
io8_ft_v33_hs_pd_3v3  "IO8_FT_V33 high speed @ 3.3V pulldown"
io8_ft_v33_fs_3v3  "IO8_FT_V33 fast speed @ 3.3V"
io8_ft_v33_fs_pu_3v3  "IO8_FT_V33 fast speed @ 3.3V pullup"
io8_ft_v33_fs_pd_3v3  "IO8_FT_V33 fast speed @ 3.3V pulldown"
io8_ft_v33_ms_3v3  "IO8_FT_V33 med speed @ 3.3V"
io8_ft_v33_ms_pu_3v3  "IO8_FT_V33 med speed @ 3.3V pullup"
io8_ft_v33_ms_pd_3v3  "IO8_FT_V33 med speed @ 3.3V pulldown"
io8_ft_v33_ls_3v3  "IO8_FT_V33 low speed @ 3.3V"
io8_ft_v33_ls_pu_3v3  "IO8_FT_V33 low speed @ 3.3V pullup"
io8_ft_v33_ls_pd_3v3  "IO8_FT_V33 low speed @ 3.3V pulldown"
[Model Selector] io8_100m_i2c_ft
io8_100m_ft_hs_1v2  "IO8_FT 100MHz high speed @ 1.2V"
io8_100m_ft_hs_pu_1v2  "IO8_FT 100MHz high speed @ 1.2V pullup"
io8_100m_ft_hs_pd_1v2  "IO8_FT 100MHz high speed @ 1.2V pulldown"
io8_100m_ft_fs_1v2  "IO8_FT 100MHz fast speed @ 1.2V"
io8_100m_ft_fs_pu_1v2  "IO8_FT 100MHz fast speed @ 1.2V pullup"
io8_100m_ft_fs_pd_1v2  "IO8_FT 100MHz fast speed @ 1.2V pulldown"
io8_100m_ft_ms_1v2  "IO8_FT 100MHz med speed @ 1.2V"
io8_100m_ft_ms_pu_1v2  "IO8_FT 100MHz med speed @ 1.2V pullup"
io8_100m_ft_ms_pd_1v2  "IO8_FT 100MHz med speed @ 1.2V pulldown"
io8_100m_ft_ls_1v2  "IO8_FT 100MHz low speed @ 1.2V"
io8_100m_ft_ls_pu_1v2  "IO8_FT 100MHz low speed @ 1.2V pullup"
io8_100m_ft_ls_pd_1v2  "IO8_FT 100MHz low speed @ 1.2V pulldown"
io8_100m_ft_hs_1v8  "IO8_FT 100MHz high speed @ 1.8V"
io8_100m_ft_hs_pu_1v8  "IO8_FT 100MHz high speed @ 1.8V pullup"
io8_100m_ft_hs_pd_1v8  "IO8_FT 100MHz high speed @ 1.8V pulldown"
io8_100m_ft_fs_1v8  "IO8_FT 100MHz fast speed @ 1.8V"
io8_100m_ft_fs_pu_1v8  "IO8_FT 100MHz fast speed @ 1.8V pullup"
io8_100m_ft_fs_pd_1v8  "IO8_FT 100MHz fast speed @ 1.8V pulldown"
io8_100m_ft_ms_1v8  "IO8_FT 100MHz med speed @ 1.8V"
io8_100m_ft_ms_pu_1v8  "IO8_FT 100MHz med speed @ 1.8V pullup"
io8_100m_ft_ms_pd_1v8  "IO8_FT 100MHz med speed @ 1.8V pulldown"
io8_100m_ft_ls_1v8  "IO8_FT 100MHz low speed @ 1.8V"
io8_100m_ft_ls_pu_1v8  "IO8_FT 100MHz low speed @ 1.8V pullup"
io8_100m_ft_ls_pd_1v8  "IO8_FT 100MHz low speed @ 1.8V pulldown"
io8_100m_ft_hs_3v3  "IO8_FT 100MHz high speed @ 3.3V"
io8_100m_ft_hs_pu_3v3  "IO8_FT 100MHz high speed @ 3.3V pullup"
io8_100m_ft_hs_pd_3v3  "IO8_FT 100MHz high speed @ 3.3V pulldown"
io8_100m_ft_fs_3v3  "IO8_FT 100MHz fast speed @ 3.3V"
io8_100m_ft_fs_pu_3v3  "IO8_FT 100MHz fast speed @ 3.3V pullup"
io8_100m_ft_fs_pd_3v3  "IO8_FT 100MHz fast speed @ 3.3V pulldown"
io8_100m_ft_ms_3v3  "IO8_FT 100MHz med speed @ 3.3V"
io8_100m_ft_ms_pu_3v3  "IO8_FT 100MHz med speed @ 3.3V pullup"
io8_100m_ft_ms_pd_3v3  "IO8_FT 100MHz med speed @ 3.3V pulldown"
io8_100m_ft_ls_3v3  "IO8_FT 100MHz low speed @ 3.3V"
io8_100m_ft_ls_pu_3v3  "IO8_FT 100MHz low speed @ 3.3V pullup"
io8_100m_ft_ls_pd_3v3  "IO8_FT 100MHz low speed @ 3.3V pulldown"
io8_100m_i2c_ft_1v2  "IO8_FT 100MHz I2C @ 1.2V"
io8_100m_i2c_ft_pu_1v2  "IO8_FT 100MHz I2C @ 1.2V pullup"
io8_100m_i2c_ft_pd_1v2  "IO8_FT 100MHz I2C @ 1.2V pulldown"
io8_100m_i2c_ft_1v8  "IO8_FT 100MHz I2C @ 1.8V"
io8_100m_i2c_ft_pu_1v8  "IO8_FT 100MHz I2C @ 1.8V pullup"
io8_100m_i2c_ft_pd_1v8  "IO8_FT 100MHz I2C @ 1,8V pulldown"
io8_100m_i2c_ft_3v3  "IO8_FT 100MHz I2C @ 3.3V"
io8_100m_i2c_ft_pu_3v3  "IO8_FT 100MHz I2C HSLV @ 3.3V pullup"
io8_100m_i2c_ft_pd_3v3  "IO8_FT 100MHz I2C @ 3.3V pulldown"
[Model Selector] io8_100m_tamp_ft
io8_100m_ft_hs_1v2  "IO8_FT 100MHz high speed @ 1.2V"
io8_100m_ft_hs_pu_1v2  "IO8_FT 100MHz high speed @ 1.2V pullup"
io8_100m_ft_hs_pd_1v2  "IO8_FT 100MHz high speed @ 1.2V pulldown"
io8_100m_ft_fs_1v2  "IO8_FT 100MHz fast speed @ 1.2V"
io8_100m_ft_fs_pu_1v2  "IO8_FT 100MHz fast speed @ 1.2V pullup"
io8_100m_ft_fs_pd_1v2  "IO8_FT 100MHz fast speed @ 1.2V pulldown"
io8_100m_ft_ms_1v2  "IO8_FT 100MHz med speed @ 1.2V"
io8_100m_ft_ms_pu_1v2  "IO8_FT 100MHz med speed @ 1.2V pullup"
io8_100m_ft_ms_pd_1v2  "IO8_FT 100MHz med speed @ 1.2V pulldown"
io8_100m_ft_ls_1v2  "IO8_FT 100MHz low speed @ 1.2V"
io8_100m_ft_ls_pu_1v2  "IO8_FT 100MHz low speed @ 1.2V pullup"
io8_100m_ft_ls_pd_1v2  "IO8_FT 100MHz low speed @ 1.2V pulldown"
io8_100m_ft_hs_1v8  "IO8_FT 100MHz high speed @ 1.8V"
io8_100m_ft_hs_pu_1v8  "IO8_FT 100MHz high speed @ 1.8V pullup"
io8_100m_ft_hs_pd_1v8  "IO8_FT 100MHz high speed @ 1.8V pulldown"
io8_100m_ft_fs_1v8  "IO8_FT 100MHz fast speed @ 1.8V"
io8_100m_ft_fs_pu_1v8  "IO8_FT 100MHz fast speed @ 1.8V pullup"
io8_100m_ft_fs_pd_1v8  "IO8_FT 100MHz fast speed @ 1.8V pulldown"
io8_100m_ft_ms_1v8  "IO8_FT 100MHz med speed @ 1.8V"
io8_100m_ft_ms_pu_1v8  "IO8_FT 100MHz med speed @ 1.8V pullup"
io8_100m_ft_ms_pd_1v8  "IO8_FT 100MHz med speed @ 1.8V pulldown"
io8_100m_ft_ls_1v8  "IO8_FT 100MHz low speed @ 1.8V"
io8_100m_ft_ls_pu_1v8  "IO8_FT 100MHz low speed @ 1.8V pullup"
io8_100m_ft_ls_pd_1v8  "IO8_FT 100MHz low speed @ 1.8V pulldown"
io8_100m_ft_hs_3v3  "IO8_FT 100MHz high speed @ 3.3V"
io8_100m_ft_hs_pu_3v3  "IO8_FT 100MHz high speed @ 3.3V pullup"
io8_100m_ft_hs_pd_3v3  "IO8_FT 100MHz high speed @ 3.3V pulldown"
io8_100m_ft_fs_3v3  "IO8_FT 100MHz fast speed @ 3.3V"
io8_100m_ft_fs_pu_3v3  "IO8_FT 100MHz fast speed @ 3.3V pullup"
io8_100m_ft_fs_pd_3v3  "IO8_FT 100MHz fast speed @ 3.3V pulldown"
io8_100m_ft_ms_3v3  "IO8_FT 100MHz med speed @ 3.3V"
io8_100m_ft_ms_pu_3v3  "IO8_FT 100MHz med speed @ 3.3V pullup"
io8_100m_ft_ms_pd_3v3  "IO8_FT 100MHz med speed @ 3.3V pulldown"
io8_100m_ft_ls_3v3  "IO8_FT 100MHz low speed @ 3.3V"
io8_100m_ft_ls_pu_3v3  "IO8_FT 100MHz low speed @ 3.3V pullup"
io8_100m_ft_ls_pd_3v3  "IO8_FT 100MHz low speed @ 3.3V pulldown"
io8_ft_v33_hs_1v2  "IO8_FT_V33 high speed @ 1.2V"
io8_ft_v33_hs_pu_1v2  "IO8_FT_V33 high speed @ 1.2V pullup"
io8_ft_v33_hs_pd_1v2  "IO8_FT_V33 high speed @ 1.2V pulldown"
io8_ft_v33_fs_1v2  "IO8_FT_V33 fast speed @ 1.2V"
io8_ft_v33_fs_pu_1v2  "IO8_FT_V33 fast speed @ 1.2V pullup"
io8_ft_v33_fs_pd_1v2  "IO8_FT_V33 fast speed @ 1.2V pulldown"
io8_ft_v33_ms_1v2  "IO8_FT_V33 med speed @ 1.2V"
io8_ft_v33_ms_pu_1v2  "IO8_FT_V33 med speed @ 1.2V pullup"
io8_ft_v33_ms_pd_1v2  "IO8_FT_V33 med speed @ 1.2V pulldown"
io8_ft_v33_ls_1v2  "IO8_FT_V33 low speed @ 1.2V"
io8_ft_v33_ls_pu_1v2  "IO8_FT_V33 low speed @ 1.2V pullup"
io8_ft_v33_ls_pd_1v2  "IO8_FT_V33 low speed @ 1.2V pulldown"
io8_ft_v33_hs_1v8  "IO8_FT_V33 high speed @ 1.8V"
io8_ft_v33_hs_pu_1v8  "IO8_FT_V33 high speed @ 1.8V pullup"
io8_ft_v33_hs_pd_1v8  "IO8_FT_V33 high speed @ 1.8V pulldown"
io8_ft_v33_fs_1v8  "IO8_FT_V33 fast speed @ 1.8V"
io8_ft_v33_fs_pu_1v8  "IO8_FT_V33 fast speed @ 1.8V pullup"
io8_ft_v33_fs_pd_1v8  "IO8_FT_V33 fast speed @ 1.8V pulldown"
io8_ft_v33_ms_1v8  "IO8_FT_V33 med speed @ 1.8V"
io8_ft_v33_ms_pu_1v8  "IO8_FT_V33 med speed @ 1.8V pullup"
io8_ft_v33_ms_pd_1v8  "IO8_FT_V33 med speed @ 1.8V pulldown"
io8_ft_v33_ls_1v8  "IO8_FT_V33 low speed @ 1.8V"
io8_ft_v33_ls_pu_1v8  "IO8_FT_V33 low speed @ 1.8V pullup"
io8_ft_v33_ls_pd_1v8  "IO8_FT_V33 low speed @ 1.8V pulldown"
io8_ft_v33_hs_3v3  "IO8_FT_V33 high speed @ 3.3V"
io8_ft_v33_hs_pu_3v3  "IO8_FT_V33 high speed @ 3.3V pullup"
io8_ft_v33_hs_pd_3v3  "IO8_FT_V33 high speed @ 3.3V pulldown"
io8_ft_v33_fs_3v3  "IO8_FT_V33 fast speed @ 3.3V"
io8_ft_v33_fs_pu_3v3  "IO8_FT_V33 fast speed @ 3.3V pullup"
io8_ft_v33_fs_pd_3v3  "IO8_FT_V33 fast speed @ 3.3V pulldown"
io8_ft_v33_ms_3v3  "IO8_FT_V33 med speed @ 3.3V"
io8_ft_v33_ms_pu_3v3  "IO8_FT_V33 med speed @ 3.3V pullup"
io8_ft_v33_ms_pd_3v3  "IO8_FT_V33 med speed @ 3.3V pulldown"
io8_ft_v33_ls_3v3  "IO8_FT_V33 low speed @ 3.3V"
io8_ft_v33_ls_pu_3v3  "IO8_FT_V33 low speed @ 3.3V pullup"
io8_ft_v33_ls_pd_3v3  "IO8_FT_V33 low speed @ 3.3V pulldown"
[Model Selector] io8_usb_ft
io8_100m_ft_hs_1v2  "IO8_FT 100MHz high speed @ 1.2V"
io8_100m_ft_hs_pu_1v2  "IO8_FT 100MHz high speed @ 1.2V pullup"
io8_100m_ft_hs_pd_1v2  "IO8_FT 100MHz high speed @ 1.2V pulldown"
io8_100m_ft_fs_1v2  "IO8_FT 100MHz fast speed @ 1.2V"
io8_100m_ft_fs_pu_1v2  "IO8_FT 100MHz fast speed @ 1.2V pullup"
io8_100m_ft_fs_pd_1v2  "IO8_FT 100MHz fast speed @ 1.2V pulldown"
io8_100m_ft_ms_1v2  "IO8_FT 100MHz med speed @ 1.2V"
io8_100m_ft_ms_pu_1v2  "IO8_FT 100MHz med speed @ 1.2V pullup"
io8_100m_ft_ms_pd_1v2  "IO8_FT 100MHz med speed @ 1.2V pulldown"
io8_100m_ft_ls_1v2  "IO8_FT 100MHz low speed @ 1.2V"
io8_100m_ft_ls_pu_1v2  "IO8_FT 100MHz low speed @ 1.2V pullup"
io8_100m_ft_ls_pd_1v2  "IO8_FT 100MHz low speed @ 1.2V pulldown"
io8_100m_ft_hs_1v8  "IO8_FT 100MHz high speed @ 1.8V"
io8_100m_ft_hs_pu_1v8  "IO8_FT 100MHz high speed @ 1.8V pullup"
io8_100m_ft_hs_pd_1v8  "IO8_FT 100MHz high speed @ 1.8V pulldown"
io8_100m_ft_fs_1v8  "IO8_FT 100MHz fast speed @ 1.8V"
io8_100m_ft_fs_pu_1v8  "IO8_FT 100MHz fast speed @ 1.8V pullup"
io8_100m_ft_fs_pd_1v8  "IO8_FT 100MHz fast speed @ 1.8V pulldown"
io8_100m_ft_ms_1v8  "IO8_FT 100MHz med speed @ 1.8V"
io8_100m_ft_ms_pu_1v8  "IO8_FT 100MHz med speed @ 1.8V pullup"
io8_100m_ft_ms_pd_1v8  "IO8_FT 100MHz med speed @ 1.8V pulldown"
io8_100m_ft_ls_1v8  "IO8_FT 100MHz low speed @ 1.8V"
io8_100m_ft_ls_pu_1v8  "IO8_FT 100MHz low speed @ 1.8V pullup"
io8_100m_ft_ls_pd_1v8  "IO8_FT 100MHz low speed @ 1.8V pulldown"
io8_100m_ft_hs_3v3  "IO8_FT 100MHz high speed @ 3.3V"
io8_100m_ft_hs_pu_3v3  "IO8_FT 100MHz high speed @ 3.3V pullup"
io8_100m_ft_hs_pd_3v3  "IO8_FT 100MHz high speed @ 3.3V pulldown"
io8_100m_ft_fs_3v3  "IO8_FT 100MHz fast speed @ 3.3V"
io8_100m_ft_fs_pu_3v3  "IO8_FT 100MHz fast speed @ 3.3V pullup"
io8_100m_ft_fs_pd_3v3  "IO8_FT 100MHz fast speed @ 3.3V pulldown"
io8_100m_ft_ms_3v3  "IO8_FT 100MHz med speed @ 3.3V"
io8_100m_ft_ms_pu_3v3  "IO8_FT 100MHz med speed @ 3.3V pullup"
io8_100m_ft_ms_pd_3v3  "IO8_FT 100MHz med speed @ 3.3V pulldown"
io8_100m_ft_ls_3v3  "IO8_FT 100MHz low speed @ 3.3V"
io8_100m_ft_ls_pu_3v3  "IO8_FT 100MHz low speed @ 3.3V pullup"
io8_100m_ft_ls_pd_3v3  "IO8_FT 100MHz low speed @ 3.3V pulldown"
io8_usb_fs_3v3  "IOUSB fast speed @ 3.3V"
io8_usb_fs_pu1_3v3  "IO8USB fast speed @ 3.3V pullup1"
io8_usb_fs_pd1_3v3  "IOUSB fast speed @ 3.3V pulldown1"
io8_usb_ls_3v3  "IOUSB low speed @ 3.3V"
io8_usb_ls_pu1_3v3  "IOUSB low speed @ 3.3V pullup1"
io8_usb_ls_pd1_3v3  "IOUSB low speed @ 3.3V pulldown1"
io8_usb_fs_pu2_3v3  "IOUSB fast speed @ 3.3V pullup2"
io8_usb_fs_pd2_3v3  "IOUSB fast speed @ 3.3V pulldown2"
io8_usb_ls_pu2_3v3  "IOUSB low speed @ 3.3V pullup2"
io8_usb_ls_pd2_3v3  "IOUSB low speed @ 3.3V pulldown2"
[Model Selector] io8_166m_hslv_ft
io8_166m_ft_hs_1v2  "IO8_FT 166MHz high speed @ 1.2V"
io8_166m_ft_hs_pu_1v2  "IO8_FT 166MHz high speed @ 1.2V pullup"
io8_166m_ft_hs_pd_1v2  "IO8_FT 166MHz high speed @ 1.2V pulldown"
io8_166m_ft_fs_1v2  "IO8_FT 166MHz fast speed @ 1.2V"
io8_166m_ft_fs_pu_1v2  "IO8_FT 166MHz fast speed @ 1.2V pullup"
io8_166m_ft_fs_pd_1v2  "IO8_FT 166MHz fast speed @ 1.2V pulldown"
io8_166m_ft_ms_1v2  "IO8_FT 166MHz med speed @ 1.2V"
io8_166m_ft_ms_pu_1v2  "IO8_FT 166MHz med speed @ 1.2V pullup"
io8_166m_ft_ms_pd_1v2  "IO8_FT 166MHz med speed @ 1.2V pulldown"
io8_166m_ft_ls_1v2  "IO8_FT 166MHz low speed @ 1.2V"
io8_166m_ft_ls_pu_1v2  "IO8_FT 166MHz low speed @ 1.2V pullup"
io8_166m_ft_ls_pd_1v2  "IO8_FT 166MHz low speed @ 1.2V pulldown"
io8_166m_ft_hs_1v8  "IO8_FT 166MHz high speed @ 1.8V"
io8_166m_ft_hs_pu_1v8  "IO8_FT 166MHz high speed @ 1.8V pullup"
io8_166m_ft_hs_pd_1v8  "IO8_FT 166MHz high speed @ 1.8V pulldown"
io8_166m_ft_fs_1v8  "IO8_FT 166MHz fast speed @ 1.8V"
io8_166m_ft_fs_pu_1v8  "IO8_FT 166MHz fast speed @ 1.8V pullup"
io8_166m_ft_fs_pd_1v8  "IO8_FT 166MHz fast speed @ 1.8V pulldown"
io8_166m_ft_ms_1v8  "IO8_FT 166MHz med speed @ 1.8V"
io8_166m_ft_ms_pu_1v8  "IO8_FT 166MHz med speed @ 1.8V pullup"
io8_166m_ft_ms_pd_1v8  "IO8_FT 166MHz med speed @ 1.8V pulldown"
io8_166m_ft_ls_1v8  "IO8_FT 166MHz low speed @ 1.8V"
io8_166m_ft_ls_pu_1v8  "IO8_FT 166MHz low speed @ 1.8V pullup"
io8_166m_ft_ls_pd_1v8  "IO8_FT 166MHz low speed @ 1.8V pulldown"
io8_166m_ft_hs_3v3  "IO8_FT 166MHz high speed @ 3.3V"
io8_166m_ft_hs_pu_3v3  "IO8_FT 166MHz high speed @ 3.3V pullup"
io8_166m_ft_hs_pd_3v3  "IO8_FT 166MHz high speed @ 3.3V pulldown"
io8_166m_ft_fs_3v3  "IO8_FT 166MHz fast speed @ 3.3V"
io8_166m_ft_fs_pu_3v3  "IO8_FT 166MHz fast speed @ 3.3V pullup"
io8_166m_ft_fs_pd_3v3  "IO8_FT 166MHz fast speed @ 3.3V pulldown"
io8_166m_ft_ms_3v3  "IO8_FT 166MHz med speed @ 3.3V"
io8_166m_ft_ms_pu_3v3  "IO8_FT 166MHz med speed @ 3.3V pullup"
io8_166m_ft_ms_pd_3v3  "IO8_FT 166MHz med speed @ 3.3V pulldown"
io8_166m_ft_ls_3v3  "IO8_FT 166MHz low speed @ 3.3V"
io8_166m_ft_ls_pu_3v3  "IO8_FT 166MHz low speed @ 3.3V pullup"
io8_166m_ft_ls_pd_3v3  "IO8_FT 166MHz low speed @ 3.3V pulldown"
io8_166m_hslv_ft_hs_1v2  "IO8_FT 166MHz HSLV high speed @ 1.2V"
io8_166m_hslv_ft_hs_pu_1v2  "IO8_FT 166MHz HSLV high speed @ 1.2V pullup"
io8_166m_hslv_ft_hs_pd_1v2  "IO8_FT 166MHz HSLV high speed @ 1.2V pulldown"
io8_166m_hslv_ft_fs_1v2  "IO8_FT 166MHz HSLV fast speed @ 1.2V"
io8_166m_hslv_ft_fs_pu_1v2  "IO8_FT 166MHz HSLV fast speed @ 1.2V pullup"
io8_166m_hslv_ft_fs_pd_1v2  "IO8_FT 166MHz HSLV fast speed @ 1.2V pulldown"
io8_166m_hslv_ft_ms_1v2  "IO8_FT 166MHz HSLV med speed @ 1.2V"
io8_166m_hslv_ft_ms_pu_1v2  "IO8_FT 166MHz HSLV med speed @ 1.2V pullup"
io8_166m_hslv_ft_ms_pd_1v2  "IO8_FT 166MHz HSLV med speed @ 1.2V pulldown"
io8_166m_hslv_ft_ls_1v2  "IO8_FT 166MHz HSLV low speed @ 1.2V"
io8_166m_hslv_ft_ls_pu_1v2  "IO8_FT 166MHz HSLV low speed @ 1.2V pullup"
io8_166m_hslv_ft_ls_pd_1v2  "IO8_FT 166MHz HSLV low speed @ 1.2V pulldown"
io8_166m_hslv_ft_hs_1v8  "IO8_FT 166MHz HSLV high speed @ 1.8V"
io8_166m_hslv_ft_hs_pu_1v8  "IO8_FT 166MHz HSLV high speed @ 1.8V pullup"
io8_166m_hslv_ft_hs_pd_1v8  "IO8_FT 166MHz HSLV high speed @ 1.8V pulldown"
io8_166m_hslv_ft_fs_1v8  "IO8_FT 166MHz HSLV fast speed @ 1.8V"
io8_166m_hslv_ft_fs_pu_1v8  "IO8_FT 166MHz HSLV fast speed @ 1.8V pullup"
io8_166m_hslv_ft_fs_pd_1v8  "IO8_FT 166MHz HSLV fast speed @ 1.8V pulldown"
io8_166m_hslv_ft_ms_1v8  "IO8_FT 166MHz HSLV med speed @ 1.8V"
io8_166m_hslv_ft_ms_pu_1v8  "IO8_FT 166MHz HSLV med speed @ 1.8V pullup"
io8_166m_hslv_ft_ms_pd_1v8  "IO8_FT 166MHz HSLV med speed @ 1.8V pulldown"
io8_166m_hslv_ft_ls_1v8  "IO8_FT 166MHz HSLV low speed @ 1.8V"
io8_166m_hslv_ft_ls_pu_1v8  "IO8_FT 166MHz HSLV low speed @ 1.8V pullup"
io8_166m_hslv_ft_ls_pd_1v8  "IO8_FT 166MHz HSLV low speed @ 1.8V pulldown"
io8_166m_hslv_ft_hs_2v5  "IO8_FT 166MHz HSLV high speed @ 2.5V"
io8_166m_hslv_ft_hs_pu_2v5  "IO8_FT 166MHz HSLV high speed @ 2.5V pullup"
io8_166m_hslv_ft_hs_pd_2v5  "IO8_FT 166MHz HSLV high speed @ 2.5V pulldown"
io8_166m_hslv_ft_fs_2v5  "IO8_FT 166MHz HSLV fast speed @ 2.5V"
io8_166m_hslv_ft_fs_pu_2v5  "IO8_FT 166MHz HSLV fast speed @ 2.5V pullup"
io8_166m_hslv_ft_fs_pd_2v5  "IO8_FT 166MHz HSLV fast speed @ 2.5V pulldown"
io8_166m_hslv_ft_ms_2v5  "IO8_FT 166MHz HSLV med speed @ 2.5V"
io8_166m_hslv_ft_ms_pu_2v5  "IO8_FT 166MHz HSLV med speed @ 2.5V pullup"
io8_166m_hslv_ft_ms_pd_2v5  "IO8_FT 166MHz HSLV med speed @ 2.5V pulldown"
io8_166m_hslv_ft_ls_2v5  "IO8_FT 166MHz HSLV low speed @ 2.5V"
io8_166m_hslv_ft_ls_pu_2v5  "IO8_FT 166MHz HSLV low speed @ 2.5V pullup"
io8_166m_hslv_ft_ls_pd_2v5  "IO8_FT 166MHz HSLV low speed @ 2.5V pulldown"
[Model Selector] io8_166m_hslv_i2c_ft
io8_166m_ft_hs_1v2  "IO8_FT 166MHz high speed @ 1.2V"
io8_166m_ft_hs_pu_1v2  "IO8_FT 166MHz high speed @ 1.2V pullup"
io8_166m_ft_hs_pd_1v2  "IO8_FT 166MHz high speed @ 1.2V pulldown"
io8_166m_ft_fs_1v2  "IO8_FT 166MHz fast speed @ 1.2V"
io8_166m_ft_fs_pu_1v2  "IO8_FT 166MHz fast speed @ 1.2V pullup"
io8_166m_ft_fs_pd_1v2  "IO8_FT 166MHz fast speed @ 1.2V pulldown"
io8_166m_ft_ms_1v2  "IO8_FT 166MHz med speed @ 1.2V"
io8_166m_ft_ms_pu_1v2  "IO8_FT 166MHz med speed @ 1.2V pullup"
io8_166m_ft_ms_pd_1v2  "IO8_FT 166MHz med speed @ 1.2V pulldown"
io8_166m_ft_ls_1v2  "IO8_FT 166MHz low speed @ 1.2V"
io8_166m_ft_ls_pu_1v2  "IO8_FT 166MHz low speed @ 1.2V pullup"
io8_166m_ft_ls_pd_1v2  "IO8_FT 166MHz low speed @ 1.2V pulldown"
io8_166m_ft_hs_1v8  "IO8_FT 166MHz high speed @ 1.8V"
io8_166m_ft_hs_pu_1v8  "IO8_FT 166MHz high speed @ 1.8V pullup"
io8_166m_ft_hs_pd_1v8  "IO8_FT 166MHz high speed @ 1.8V pulldown"
io8_166m_ft_fs_1v8  "IO8_FT 166MHz fast speed @ 1.8V"
io8_166m_ft_fs_pu_1v8  "IO8_FT 166MHz fast speed @ 1.8V pullup"
io8_166m_ft_fs_pd_1v8  "IO8_FT 166MHz fast speed @ 1.8V pulldown"
io8_166m_ft_ms_1v8  "IO8_FT 166MHz med speed @ 1.8V"
io8_166m_ft_ms_pu_1v8  "IO8_FT 166MHz med speed @ 1.8V pullup"
io8_166m_ft_ms_pd_1v8  "IO8_FT 166MHz med speed @ 1.8V pulldown"
io8_166m_ft_ls_1v8  "IO8_FT 166MHz low speed @ 1.8V"
io8_166m_ft_ls_pu_1v8  "IO8_FT 166MHz low speed @ 1.8V pullup"
io8_166m_ft_ls_pd_1v8  "IO8_FT 166MHz low speed @ 1.8V pulldown"
io8_166m_ft_hs_3v3  "IO8_FT 166MHz high speed @ 3.3V"
io8_166m_ft_hs_pu_3v3  "IO8_FT 166MHz high speed @ 3.3V pullup"
io8_166m_ft_hs_pd_3v3  "IO8_FT 166MHz high speed @ 3.3V pulldown"
io8_166m_ft_fs_3v3  "IO8_FT 166MHz fast speed @ 3.3V"
io8_166m_ft_fs_pu_3v3  "IO8_FT 166MHz fast speed @ 3.3V pullup"
io8_166m_ft_fs_pd_3v3  "IO8_FT 166MHz fast speed @ 3.3V pulldown"
io8_166m_ft_ms_3v3  "IO8_FT 166MHz med speed @ 3.3V"
io8_166m_ft_ms_pu_3v3  "IO8_FT 166MHz med speed @ 3.3V pullup"
io8_166m_ft_ms_pd_3v3  "IO8_FT 166MHz med speed @ 3.3V pulldown"
io8_166m_ft_ls_3v3  "IO8_FT 166MHz low speed @ 3.3V"
io8_166m_ft_ls_pu_3v3  "IO8_FT 166MHz low speed @ 3.3V pullup"
io8_166m_ft_ls_pd_3v3  "IO8_FT 166MHz low speed @ 3.3V pulldown"
io8_166m_hslv_ft_hs_1v2  "IO8_FT 166MHz HSLV high speed @ 1.2V"
io8_166m_hslv_ft_hs_pu_1v2  "IO8_FT 166MHz HSLV high speed @ 1.2V pullup"
io8_166m_hslv_ft_hs_pd_1v2  "IO8_FT 166MHz HSLV high speed @ 1.2V pulldown"
io8_166m_hslv_ft_fs_1v2  "IO8_FT 166MHz HSLV fast speed @ 1.2V"
io8_166m_hslv_ft_fs_pu_1v2  "IO8_FT 166MHz HSLV fast speed @ 1.2V pullup"
io8_166m_hslv_ft_fs_pd_1v2  "IO8_FT 166MHz HSLV fast speed @ 1.2V pulldown"
io8_166m_hslv_ft_ms_1v2  "IO8_FT 166MHz HSLV med speed @ 1.2V"
io8_166m_hslv_ft_ms_pu_1v2  "IO8_FT 166MHz HSLV med speed @ 1.2V pullup"
io8_166m_hslv_ft_ms_pd_1v2  "IO8_FT 166MHz HSLV med speed @ 1.2V pulldown"
io8_166m_hslv_ft_ls_1v2  "IO8_FT 166MHz HSLV low speed @ 1.2V"
io8_166m_hslv_ft_ls_pu_1v2  "IO8_FT 166MHz HSLV low speed @ 1.2V pullup"
io8_166m_hslv_ft_ls_pd_1v2  "IO8_FT 166MHz HSLV low speed @ 1.2V pulldown"
io8_166m_hslv_ft_hs_1v8  "IO8_FT 166MHz HSLV high speed @ 1.8V"
io8_166m_hslv_ft_hs_pu_1v8  "IO8_FT 166MHz HSLV high speed @ 1.8V pullup"
io8_166m_hslv_ft_hs_pd_1v8  "IO8_FT 166MHz HSLV high speed @ 1.8V pulldown"
io8_166m_hslv_ft_fs_1v8  "IO8_FT 166MHz HSLV fast speed @ 1.8V"
io8_166m_hslv_ft_fs_pu_1v8  "IO8_FT 166MHz HSLV fast speed @ 1.8V pullup"
io8_166m_hslv_ft_fs_pd_1v8  "IO8_FT 166MHz HSLV fast speed @ 1.8V pulldown"
io8_166m_hslv_ft_ms_1v8  "IO8_FT 166MHz HSLV med speed @ 1.8V"
io8_166m_hslv_ft_ms_pu_1v8  "IO8_FT 166MHz HSLV med speed @ 1.8V pullup"
io8_166m_hslv_ft_ms_pd_1v8  "IO8_FT 166MHz HSLV med speed @ 1.8V pulldown"
io8_166m_hslv_ft_ls_1v8  "IO8_FT 166MHz HSLV low speed @ 1.8V"
io8_166m_hslv_ft_ls_pu_1v8  "IO8_FT 166MHz HSLV low speed @ 1.8V pullup"
io8_166m_hslv_ft_ls_pd_1v8  "IO8_FT 166MHz HSLV low speed @ 1.8V pulldown"
io8_166m_hslv_ft_hs_2v5  "IO8_FT 166MHz HSLV high speed @ 2.5V"
io8_166m_hslv_ft_hs_pu_2v5  "IO8_FT 166MHz HSLV high speed @ 2.5V pullup"
io8_166m_hslv_ft_hs_pd_2v5  "IO8_FT 166MHz HSLV high speed @ 2.5V pulldown"
io8_166m_hslv_ft_fs_2v5  "IO8_FT 166MHz HSLV fast speed @ 2.5V"
io8_166m_hslv_ft_fs_pu_2v5  "IO8_FT 166MHz HSLV fast speed @ 2.5V pullup"
io8_166m_hslv_ft_fs_pd_2v5  "IO8_FT 166MHz HSLV fast speed @ 2.5V pulldown"
io8_166m_hslv_ft_ms_2v5  "IO8_FT 166MHz HSLV med speed @ 2.5V"
io8_166m_hslv_ft_ms_pu_2v5  "IO8_FT 166MHz HSLV med speed @ 2.5V pullup"
io8_166m_hslv_ft_ms_pd_2v5  "IO8_FT 166MHz HSLV med speed @ 2.5V pulldown"
io8_166m_hslv_ft_ls_2v5  "IO8_FT 166MHz HSLV low speed @ 2.5V"
io8_166m_hslv_ft_ls_pu_2v5  "IO8_FT 166MHz HSLV low speed @ 2.5V pullup"
io8_166m_hslv_ft_ls_pd_2v5  "IO8_FT 166MHz HSLV low speed @ 2.5V pulldown"
io8_166m_i2c_ft_1v2  "IO8_FT 166MHz I2C @ 1.2V"
io8_166m_i2c_ft_pu_1v2  "IO8_FT 166MHz I2C @ 1.2V pullup"
io8_166m_i2c_ft_pd_1v2  "IO8_FT 166MHz I2C @ 1.2V pulldown"
io8_166m_i2c_ft_1v8  "IO8_FT 166MHz I2C @ 1.8V"
io8_166m_i2c_ft_pu_1v8  "IO8_FT 166MHz I2C @ 1.8V pullup"
io8_166m_i2c_ft_pd_1v8  "IO8_FT 166MHz I2C @ 1,8V pulldown"
io8_166m_i2c_ft_3v3  "IO8_FT 166MHz I2C @ 3.3V"
io8_166m_i2c_ft_pu_3v3  "IO8_FT 166MHz I2C HSLV @ 3.3V pullup"
io8_166m_i2c_ft_pd_3v3  "IO8_FT 166MHz I2C @ 3.3V pulldown"
[Model Selector] io8_100m_ft_v33
io8_ft_v33_hs_1v2  "IO8_FT_V33 high speed @ 1.2V"
io8_ft_v33_hs_pu_1v2  "IO8_FT_V33 high speed @ 1.2V pullup"
io8_ft_v33_hs_pd_1v2  "IO8_FT_V33 high speed @ 1.2V pulldown"
io8_ft_v33_fs_1v2  "IO8_FT_V33 fast speed @ 1.2V"
io8_ft_v33_fs_pu_1v2  "IO8_FT_V33 fast speed @ 1.2V pullup"
io8_ft_v33_fs_pd_1v2  "IO8_FT_V33 fast speed @ 1.2V pulldown"
io8_ft_v33_ms_1v2  "IO8_FT_V33 med speed @ 1.2V"
io8_ft_v33_ms_pu_1v2  "IO8_FT_V33 med speed @ 1.2V pullup"
io8_ft_v33_ms_pd_1v2  "IO8_FT_V33 med speed @ 1.2V pulldown"
io8_ft_v33_ls_1v2  "IO8_FT_V33 low speed @ 1.2V"
io8_ft_v33_ls_pu_1v2  "IO8_FT_V33 low speed @ 1.2V pullup"
io8_ft_v33_ls_pd_1v2  "IO8_FT_V33 low speed @ 1.2V pulldown"
io8_ft_v33_hs_1v8  "IO8_FT_V33 high speed @ 1.8V"
io8_ft_v33_hs_pu_1v8  "IO8_FT_V33 high speed @ 1.8V pullup"
io8_ft_v33_hs_pd_1v8  "IO8_FT_V33 high speed @ 1.8V pulldown"
io8_ft_v33_fs_1v8  "IO8_FT_V33 fast speed @ 1.8V"
io8_ft_v33_fs_pu_1v8  "IO8_FT_V33 fast speed @ 1.8V pullup"
io8_ft_v33_fs_pd_1v8  "IO8_FT_V33 fast speed @ 1.8V pulldown"
io8_ft_v33_ms_1v8  "IO8_FT_V33 med speed @ 1.8V"
io8_ft_v33_ms_pu_1v8  "IO8_FT_V33 med speed @ 1.8V pullup"
io8_ft_v33_ms_pd_1v8  "IO8_FT_V33 med speed @ 1.8V pulldown"
io8_ft_v33_ls_1v8  "IO8_FT_V33 low speed @ 1.8V"
io8_ft_v33_ls_pu_1v8  "IO8_FT_V33 low speed @ 1.8V pullup"
io8_ft_v33_ls_pd_1v8  "IO8_FT_V33 low speed @ 1.8V pulldown"
io8_ft_v33_hs_3v3  "IO8_FT_V33 high speed @ 3.3V"
io8_ft_v33_hs_pu_3v3  "IO8_FT_V33 high speed @ 3.3V pullup"
io8_ft_v33_hs_pd_3v3  "IO8_FT_V33 high speed @ 3.3V pulldown"
io8_ft_v33_fs_3v3  "IO8_FT_V33 fast speed @ 3.3V"
io8_ft_v33_fs_pu_3v3  "IO8_FT_V33 fast speed @ 3.3V pullup"
io8_ft_v33_fs_pd_3v3  "IO8_FT_V33 fast speed @ 3.3V pulldown"
io8_ft_v33_ms_3v3  "IO8_FT_V33 med speed @ 3.3V"
io8_ft_v33_ms_pu_3v3  "IO8_FT_V33 med speed @ 3.3V pullup"
io8_ft_v33_ms_pd_3v3  "IO8_FT_V33 med speed @ 3.3V pulldown"
io8_ft_v33_ls_3v3  "IO8_FT_V33 low speed @ 3.3V"
io8_ft_v33_ls_pu_3v3  "IO8_FT_V33 low speed @ 3.3V pullup"
io8_ft_v33_ls_pd_3v3  "IO8_FT_V33 low speed @ 3.3V pulldown"
[Define Package Model]  455-ufbga-7x7-100-smps-100mhz-230421
[Manufacturer]  unknown
[OEM]  unknown
[Description]  unknown
[Number Of Pins]  92
[Pin Numbers]
| Pin Name Terminal   Net Name   Starting Node   Ending Node
F1 | NRST
J3 | PA0
J2 | PA1
K1 | PA2
K2 | PA3
L1 | PA4
L2 | PA5
M1 | PA6
M2 | PA7
F12 | PA8
E11 | PA9
E12 | PA10
D12 | PA11
D11 | PA12
C12 | PA13
C11 | PA14
B12 | PA15
L3 | PB0
M3 | PB1
L4 | PB2
B6 | PB3
A6 | PB4
B5 | PB5
A5 | PB6
A4 | PB7
B4 | PB8
A1 | PB9
M8 | PB10
K8 | PB11
L11 | PB13
M11 | PB14
M12 | PB15
F2 | PC0
G1 | PC1
G2 | PC2
H3 | PC3
H12 | PC6
G11 | PC7
G12 | PC8
F11 | PC9
A12 | PC10
B11 | PC11
C9 | PC12
E3 | PC13
D1 | PC14-OSC32_IN
D2 | PC15-OSC32_OUT
A11 | PD0
B10 | PD1
A10 | PD2
B9 | PD3
A9 | PD4
A8 | PD5
B8 | PD6
A7 | PD7
J10 | PD8
K11 | PD9
L12 | PD10
K12 | PD11
H10 | PD12
J11 | PD13
J12 | PD14
H11 | PD15
A2 | PE0
B1 | PE2
B2 | PE3
B3 | PE4
D3 | PE5
C2 | PE6
K5 | PE7
M4 | PE8
L5 | PE9
M5 | PE10
L6 | PE11
M6 | PE12
L7 | PE13
M7 | PE14
L8 | PE15
E1 | PH0-OSC_IN
E2 | PH1-OSC_OUT
A3 | PH3-BOOT0
K9 | VDD11
C5 | VDD11
C1 | VBAT
B7 | VDD
J1 | VDDA
M10 | VDDSMPS
E10 | VDDUSB
M9 | VLXSMPS
H1 | VREFP
C4 | VSS
H2 | VSSA
L9 | VSSSMPS
|[Merged Pins]  C4
|C8  |  VSS
|D10  |  VSS
|K3  |  VSS
|L10  |  VSS
|[Merged Pins]  B7
|C3  |  VDD
|C10  |  VDD
|K4  |  VDD
|K10  |  VDD
[Model Data]
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[End Model Data]
[End Package Model]
| Models and submodels in the file (208): io8_100m_ft_hs_1v2 (I/O), io8_100m_ft_hs_pu_1v2 (I/O), io8_100m_ft_hs_pd_1v2 (I/O), io8_100m_ft_fs_1v2 (I/O), io8_100m_ft_fs_pu_1v2 (I/O), io8_100m_ft_fs_pd_1v2 (I/O), io8_100m_ft_ms_1v2 (I/O), io8_100m_ft_ms_pu_1v2 (I/O), io8_100m_ft_ms_pd_1v2 (I/O), io8_100m_ft_ls_1v2 (I/O), io8_100m_ft_ls_pu_1v2 (I/O), io8_100m_ft_ls_pd_1v2 (I/O), io8_100m_ft_hs_1v8 (I/O), io8_100m_ft_hs_pu_1v8 (I/O), io8_100m_ft_hs_pd_1v8 (I/O), io8_100m_ft_fs_1v8 (I/O), io8_100m_ft_fs_pu_1v8 (I/O), io8_100m_ft_fs_pd_1v8 (I/O), io8_100m_ft_ms_1v8 (I/O), io8_100m_ft_ms_pu_1v8 (I/O), io8_100m_ft_ms_pd_1v8 (I/O), io8_100m_ft_ls_1v8 (I/O), io8_100m_ft_ls_pu_1v8 (I/O), io8_100m_ft_ls_pd_1v8 (I/O), io8_100m_ft_hs_3v3 (I/O), io8_100m_ft_hs_pu_3v3 (I/O), io8_100m_ft_hs_pd_3v3 (I/O), io8_100m_ft_fs_3v3 (I/O), io8_100m_ft_fs_pu_3v3 (I/O), io8_100m_ft_fs_pd_3v3 (I/O), io8_100m_ft_ms_3v3 (I/O), io8_100m_ft_ms_pu_3v3 (I/O), io8_100m_ft_ms_pd_3v3 (I/O), io8_100m_ft_ls_3v3 (I/O), io8_100m_ft_ls_pu_3v3 (I/O), io8_100m_ft_ls_pd_3v3 (I/O), io8_100m_hslv_ft_hs_1v2 (I/O), io8_100m_hslv_ft_hs_pu_1v2 (I/O), io8_100m_hslv_ft_hs_pd_1v2 (I/O), io8_100m_hslv_ft_fs_1v2 (I/O), io8_100m_hslv_ft_fs_pu_1v2 (I/O), io8_100m_hslv_ft_fs_pd_1v2 (I/O), io8_100m_hslv_ft_ms_1v2 (I/O), io8_100m_hslv_ft_ms_pu_1v2 (I/O), io8_100m_hslv_ft_ms_pd_1v2 (I/O), io8_100m_hslv_ft_ls_1v2 (I/O), io8_100m_hslv_ft_ls_pu_1v2 (I/O), io8_100m_hslv_ft_ls_pd_1v2 (I/O), io8_100m_hslv_ft_hs_1v8 (I/O), io8_100m_hslv_ft_hs_pu_1v8 (I/O), io8_100m_hslv_ft_hs_pd_1v8 (I/O), io8_100m_hslv_ft_fs_1v8 (I/O), io8_100m_hslv_ft_fs_pu_1v8 (I/O), io8_100m_hslv_ft_fs_pd_1v8 (I/O), io8_100m_hslv_ft_ms_1v8 (I/O), io8_100m_hslv_ft_ms_pu_1v8 (I/O), io8_100m_hslv_ft_ms_pd_1v8 (I/O), io8_100m_hslv_ft_ls_1v8 (I/O), io8_100m_hslv_ft_ls_pu_1v8 (I/O), io8_100m_hslv_ft_ls_pd_1v8 (I/O), io8_100m_hslv_ft_hs_2v5 (I/O), io8_100m_hslv_ft_hs_pu_2v5 (I/O), io8_100m_hslv_ft_hs_pd_2v5 (I/O), io8_100m_hslv_ft_fs_2v5 (I/O), io8_100m_hslv_ft_fs_pu_2v5 (I/O), io8_100m_hslv_ft_fs_pd_2v5 (I/O), io8_100m_hslv_ft_ms_2v5 (I/O), io8_100m_hslv_ft_ms_pu_2v5 (I/O), io8_100m_hslv_ft_ms_pd_2v5 (I/O), io8_100m_hslv_ft_ls_2v5 (I/O), io8_100m_hslv_ft_ls_pu_2v5 (I/O), io8_100m_hslv_ft_ls_pd_2v5 (I/O), io8_166m_ft_hs_1v2 (I/O), io8_166m_ft_hs_pu_1v2 (I/O), io8_166m_ft_hs_pd_1v2 (I/O), io8_166m_ft_fs_1v2 (I/O), io8_166m_ft_fs_pu_1v2 (I/O), io8_166m_ft_fs_pd_1v2 (I/O), io8_166m_ft_ms_1v2 (I/O), io8_166m_ft_ms_pu_1v2 (I/O)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
